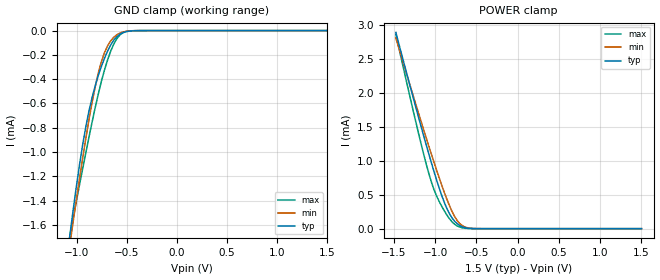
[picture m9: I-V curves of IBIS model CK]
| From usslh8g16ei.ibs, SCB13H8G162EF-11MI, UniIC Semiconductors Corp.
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|   Model CK
[Model] CK
Model_type Input
Polarity   Non-Inverting
Enable   Active-High
Vinl =  0.615V
Vinh =  0.885V
C_comp   95.580fF   78.862fF   0.112pF
C_comp_power_clamp   27.752fF   23.442fF   31.390fF
C_comp_gnd_clamp   20.038fF   15.989fF   24.661fF
[Model Spec]
Vinh   0.885V   0.776V   0.922V
Vinl   0.615V   0.506V   0.652V
[Temperature Range]   45.000   95.000   -40.000
[Voltage Range]   1.500V   1.283V   1.575V
[C Comp Corner]
C_comp_power_clamp   27.752fF   23.442fF   31.390fF
C_comp_gnd_clamp   20.038fF   15.989fF   24.661fF
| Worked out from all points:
|   GND clamp passes 1 mA (typ) near -0.95 V on its own axis
|   POWER clamp passes 1 mA (typ) near -1.05 V on its own axis
[GND_clamp]
|Voltage   I(typ)   I(min)   I(max)
-1.5V     -4.711mA   -4.355mA   -5.13mA
-1.066V   -1.656mA   -1.736mA   -1.672mA
-1.035V   -1.461mA   -1.559mA   -1.532mA
-942mV    -937.4uA   -1.048mA   -1.135mA
-849mV    -553.6uA   -594.1uA   -756.1uA
-787mV    -372.4uA   -351.5uA   -524.2uA
-725mV    -228.7uA   -182.7uA   -326uA
-663mV    -119.4uA   -85.26uA   -170.5uA
-601mV    -49.82uA   -34.44uA   -66.38uA
-539mV    -16.69uA   -11.31uA   -17.4uA
-446mV    -2.393uA   -1.69uA    -1.298uA
1.5V      0A         0A         0A
[POWER_clamp]
|Voltage   I(typ)   I(min)   I(max)
-1.476V   2.894mA    2.812mA    2.865mA
-1.197V   1.625mA    1.687mA    1.386mA
-1.104V   1.219mA    1.323mA    935.8uA
-1.042V   957.4uA    1.086mA    675.5uA
-980mV    709.1uA    854.8uA    475.2uA
-887mV    381.5uA    528.9uA    259.3uA
-825mV    216.9uA    335.6uA    144.5uA
-763mV    108.7uA    177.7uA    64.17uA
-732mV    72.5uA     118.4uA    39.23uA
-670mV    26.52uA    43.96uA    12.12uA
-546mV    1.464uA    3.136uA    422.4nA
1.5V      0A         0A         0A
